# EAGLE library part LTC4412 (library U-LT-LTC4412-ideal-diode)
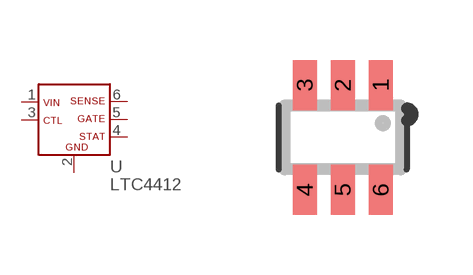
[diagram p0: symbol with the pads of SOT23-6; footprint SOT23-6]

Designator prefix U

## LTC4412  [SOT23-6]
1  VIN  pwr
2  GND  pwr
3  CTL  in
4  STAT  oc
5  GATE  out
6  SENSE  in

## Footprint SOT23-6 (pad centres in mm)
SOT23-6 Small Outline Transistor 6-pin package, 0.95 mm pitch TI DBV (R-PDSO-G5) (Falls within JEDEC MO-178 variation AA) Using 1.25 x 0.6 mm pads, mask clearance 0.07 mm, paste inset 0.025 mm.
smd 0.6 x 1.25: 1 0.95,1.31; 2 0,1.31; 3 -0.95,1.31; 4 -0.95,-1.31; 5 0,-1.31; 6 0.95,-1.31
